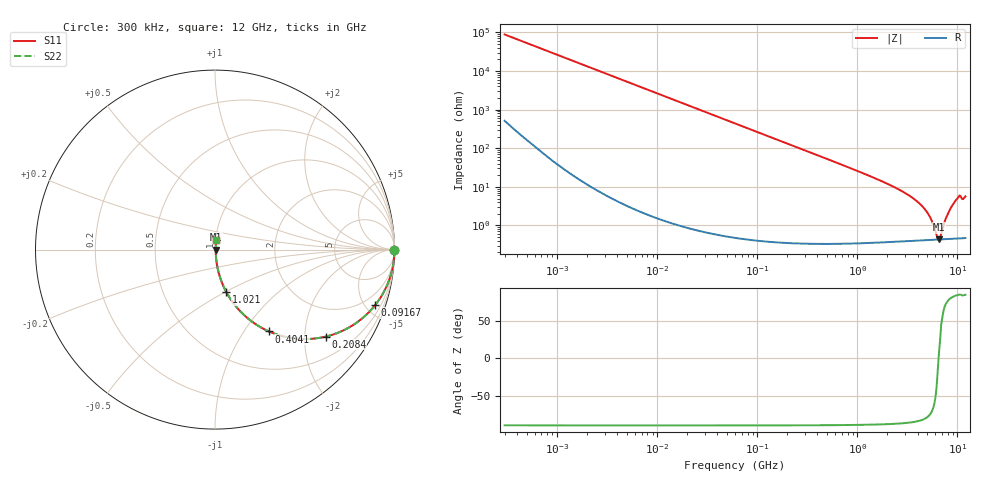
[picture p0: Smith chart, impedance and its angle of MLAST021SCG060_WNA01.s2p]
! MLAST021SCG060_WNA01  S-PARAMETER MODEL  ( General Type )
! Model Generated by TAIYO YUDEN Corporation (http://www.ty-top.com)
! Version 1.0
! TAIYO YUDEN Control No. 220901
! Copyright(c) 2022 TAIYO YUDEN CO.,LTD. All Rights Reserved.
! Product Description (link to TY-COMPAS)
! https://ds.yuden.co.jp/TYCOMPAS/or/detail?pn=MLAST021SCG060CWNA01&u=M
! Products Name : Multilayer Ceramic Capacitors
! Characteristics :
!  Capacitance : 6 pF , Rated Voltage : 25V , TCC : CG / C0G
!  Case Size : 0.25 x 0.125 / 0.0098 x 0.0049 [mm/inch] , Thickness : 0.125 / 0.0049 [mm/inch]
!  (Conditions: Temperature = 25 degC , DC Bias Current/Voltage = 0A / 0V)
! External Node Assignments :
!  1  o---| |---o  2
! GND o---------o GND
! Frequency Range : 0.3MHz  -  12000MHz  [ 401 STEP ]
# MHz S RI R 50
! Freq[MHz].  S11 Real  S11 Imag  S21 Real  S21 Imag  S12 Real  S12 Imag  S22 Real  S22 Imag
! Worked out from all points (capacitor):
!   401 points, 300 kHz to 12 GHz, reference 50 ohm
!   read as one part in series: C = 6 pF near 316.3 kHz
!   lowest |Z| = 438 mohm at 6.525 GHz (marker M1)
!   series resonance near 6.479 GHz, so ESL is about 100 pH
!   S11 on the Smith chart (normalised r, x): 300 kHz: open; 91.67 MHz: 1.01, -5.79; 208.4 MHz: 1.01, -2.54; 404.1 MHz: 1.01, -1.31; 1.021 GHz: 1.01, -0.51; 12 GHz: 1.01, +0.11
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0.3  1 -0.00113  7.85e-06 0.00113  7.85e-06 0.00113  1 -0.00113
1.769972  0.9999 -0.00667  5.08e-05 0.00667  5.08e-05 0.00667  0.9999 -0.00667
10.44266  0.9984 -0.0393  0.00157 0.0393  0.00157 0.0393  0.9984 -0.0393
27.82928  0.989 -0.1038  0.011 0.1038  0.011 0.1038  0.989 -0.1038
60  0.9511 -0.2151  0.0489 0.2151  0.0489 0.2151  0.9511 -0.2151
91.67136  0.8929 -0.3085  0.1071 0.3085  0.1071 0.3085  0.8929 -0.3085
208.3979  0.6175 -0.4846  0.3825 0.4846  0.3825 0.4846  0.6175 -0.4846
353.9943  0.3588 -0.4774  0.6412 0.4774  0.6412 0.4774  0.3588 -0.4774
404.1309  0.3004 -0.4559  0.6996 0.4559  0.6996 0.4559  0.3004 -0.4559
634.0297  0.1485 -0.3516  0.8515 0.3516  0.8515 0.3516  0.1485 -0.3516
1021.415  0.0631 -0.2364  0.9369 0.2364  0.9369 0.2364  0.0631 -0.2364
2088.533  0.0163 -0.1114  0.9837 0.1114  0.9837 0.1114  0.0163 -0.1114
3276.641  0.00749 -0.0594  0.9925 0.0594  0.9925 0.0594  0.00749 -0.0594
4385.161  0.00515 -0.0323  0.9949 0.0323  0.9949 0.0323  0.00515 -0.0323
5278.635  0.00448 -0.0165  0.9955 0.0165  0.9955 0.0165  0.00448 -0.0165
6188.031  0.00432 -0.00341  0.9957 0.00341  0.9957 0.00341  0.00432 -0.00341
6524.734  0.00434 0.000464  0.9957 -0.000464  0.9957 -0.000464  0.00434 0.000464
6879.757  0.00439 0.00439  0.9956 -0.00439  0.9956 -0.00439  0.00439 0.00439
8064.993  0.00487 0.0201  0.9951 -0.0201  0.9951 -0.0201  0.00487 0.0201
9207.246  0.00595 0.0374  0.9941 -0.0374  0.9941 -0.0374  0.00595 0.0374
10236.47  0.00748 0.0535  0.9925 -0.0535  0.9925 -0.0535  0.00748 0.0535
12000  0.00783 0.0558  0.9922 -0.0558  0.9922 -0.0558  0.00783 0.0558
